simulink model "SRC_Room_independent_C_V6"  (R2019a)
settings: Solver=VariableStepAuto  StartTime=0.0  StopTime=tend  RelTol=1e-6
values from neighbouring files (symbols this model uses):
  initial_switch = zeros(5,1)    [Main_delay.m]
  K_amb = 1    [Main_delay.m]
  K_cw = -10    [Main_delay.m]
  K_eh = 8    [Main_delay.m]
  K_hw = 12    [Main_delay.m]
  K_rw = -5    [Main_delay.m]
  Kc_CW = 1/K_cw*tau_cw/(tauC2+theta_cw)    (= -0.25)    [Main_delay.m]
  Kc_EH = 1/K_eh*tau_eh/(tauC4+theta_eh)    (= 0.3125)    [Main_delay.m]
  Kc_HW = 1/K_hw*tau_hw/(tauC3+theta_hw)    (= 0.138888888889)    [Main_delay.m]
  Kc_RW = 1/K_rw*tau_rw/(tauC1+theta_rw)    (= -0.4)    [Main_delay.m]
  KI_RW = Kc_RW/tau_I_RW    [Main_delay.m]
  Tamb0 = 18    [Main_delay.m]
  Tamb1 = 2    [Main_delay.m]
  Tamb2 = 9    [Main_delay.m]
  Tamb3 = -5    [Main_delay.m]
  Tamb4 = -25    [Main_delay.m]
  Tamb5 = 18    [Main_delay.m]
  Tamb6 = 5    [Main_delay.m]
  tau_amb = 15    [Main_delay.m]
  tau_cw = 15    [Main_delay.m]
  tau_eh = 5    [Main_delay.m]
  tau_hw = 10    [Main_delay.m]
  tau_I_CW = min(tau_cw,4*(tauC2+theta_cw))    [Main_delay.m]
  tau_I_EH = min(tau_eh,4*(tauC4+theta_eh))    [Main_delay.m]
  tau_I_HW = min(tau_hw,4*(tauC3+theta_hw))    [Main_delay.m]
  tau_I_RW = min(tau_rw,4*(tauC1+theta_rw))    [Main_delay.m]
  tau_rw = 8    [Main_delay.m]
  theta_amb = 6    [Main_delay.m]
  theta_cw = 3    [Main_delay.m]
  theta_eh = 1    [Main_delay.m]
  theta_hw = 3    [Main_delay.m]
  theta_rw = 2    [Main_delay.m]
  Tr0 = 18    [Main_delay.m]
  Tsp0 = 18    [Main_delay.m]
  Tsp1 = 0    [Main_delay.m]
  Tsp2 = 0    [Main_delay.m]
  Tsp3 = 0    [Main_delay.m]
  Tsp4 = 0    [Main_delay.m]
  Tt_CW = 1    [Main_delay.m]
  Tt_EH = 1    [Main_delay.m]
  Tt_HW = 1    [Main_delay.m]
  Tt_RW = 1    [Main_delay.m]
  tTamb1 = tTsp1    (= 10)    [Main_delay.m]
  tTamb2 = 80    [Main_delay.m]
  tTamb3 = 140    [Main_delay.m]
  tTamb4 = 180    [Main_delay.m]
  tTamb5 = 280    [Main_delay.m]
  tTamb6 = 350    [Main_delay.m]
  tTsp1 = 10    [Main_delay.m]
  tTsp2 = tTsp1+40    (= 50)    [Main_delay.m]
  tTsp3 = tTsp2+40    (= 90)    [Main_delay.m]
  tTsp4 = tTsp3+40    (= 130)    [Main_delay.m]
  v1max = 1    [Main_delay.m]
  v1min = 0    [Main_delay.m]
  v2max = 1    [Main_delay.m]
  v2min = 0    [Main_delay.m]
  v3max = 1    [Main_delay.m]
  v3min = 0    [Main_delay.m]
  v4max = 1    [Main_delay.m]
  v4min = 0    [Main_delay.m]
libraries: simulink x1

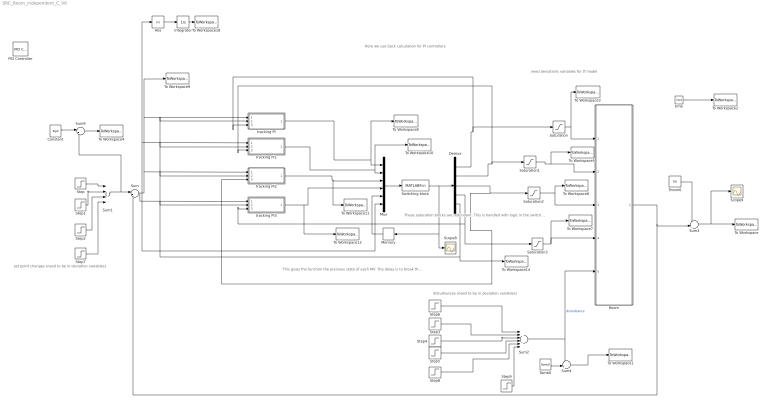
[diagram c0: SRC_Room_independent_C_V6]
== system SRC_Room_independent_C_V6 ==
  note: Here we use back calculation for PI controllers
  note: disturbances (need to be in deviation variables)
  note: set point changes (need to be in deviation variables)
  note: need deviations variables for tf model
  note: This gives the function the preivous state of each MV. The delay is to break the algebraic loop.
  note: These saturation blocks are redundant. This is handled with logic in the switching block.
  Abs : Abs
  Constant : Constant  Value=Tsp0
  Demux : Demux  Outputs=5
  Integrator : Integrator
  Memory : Memory  InitialCondition=initial_switch  InheritSampleTime=on
  Mux : Mux  Inputs=6
  PID Controller : simulink/Continuous/PID Controller  Controller=PI  Form=Parallel  TimeDomain=Continuous-time  SampleTime=-1  IntegratorMethod=Forward Euler  FilterMethod=Forward Euler  ControllerParametersSource=internal  P=Kc_RW  I=KI_RW  D=0  UseFilter=on  N=100  TunerSelectOption=Transfer Function Based (PID Tuner App)  InitialConditionSource=internal  InitialConditionForIntegrator=0  InitialConditionForFilter=0  DifferentiatorICPrevScaledInput=0  ExternalReset=none  TrackingMode=on  Kt=1  LimitOutput=off  UpperSaturationLimit=inf  LowerSaturationLimit=-inf  LinearizeAsGain=on  AntiWindupMode=none  Kb=1  POutMin=[]  POutMax=[]  IOutMin=[]  IOutMax=[]  DOutMin=[]  DOutMax=[]  NOutMin=[]  NOutMax=[]  SumOutMin=[]  SumOutMax=[]  SaturationOutMin=[]  SaturationOutMax=[]  PParamMin=[]  PParamMax=[]  IParamMin=[]  IParamMax=[]  DParamMin=[]  DParamMax=[]  NParamMin=[]  NParamMax=[]  KbParamMin=[]  KbParamMax=[]  KtParamMin=[]  KtParamMax=[]  KbOutMin=[]  KbOutMax=[]  KtOutMin=[]  KtOutMax=[]  IntegratorOutMin=[]  IntegratorOutMax=[]  FilterOutMin=[]  FilterOutMax=[]  SumI1OutMin=[]  SumI1OutMax=[]  SumI2OutMin=[]  SumI2OutMax=[]  SumI3OutMin=[]  SumI3OutMax=[]  SumI4OutMin=[]  SumI4OutMax=[]  SumDOutMin=[]  SumDOutMax=[]  DifferentiatorOutMin=[]  DifferentiatorOutMax=[]  FilterDiffOutCoefMin=[]  FilterDiffOutCoefMax=[]  ReciprocalOutMin=[]  ReciprocalOutMax=[]  SumDenOutMin=[]  SumDenOutMax=[]  SumNumOutMin=[]  SumNumOutMax=[]  DivideOutMin=[]  DivideOutMax=[]  IntegratorContinuousStateAttributes=''  IntegratorStateMustResolveToSignalObject=off  IntegratorRTWStateStorageClass=Auto  FilterContinuousStateAttributes=''  FilterStateMustResolveToSignalObject=off  FilterRTWStateStorageClass=Auto  ParallelPVariant=InternalParameters  IdealPVariant=Disabled  IVariant=InternalParameters  DVariant=Disabled  IntegratorVariant=Continuous  SatVariant=Disabled  AWVariant=Passthrough  PCopyVariant=Disabled  TRVariant=Enabled  FdbkBlocksVariant=Forward  IdealPFdbkVariant=Disabled  SatFdbkVariant=Disabled  DerivativeFilterVariant=Disabled  NVariant=Disabled  NCopyVariant=Disabled_SignalSpec  FilterICVariant=Disabled  IntegratorICVariant=InternalICs  ExternalResetVariant=Disabled  TRSumVariant=TrackingMode  SumFdbkVariant=Disabled  SumVariant=Sum_PI
  Room : Subsystem
  Saturation : Saturate  UpperLimit=v1max  LowerLimit=v1min  ZeroCross=off
  Saturation1 : Saturate  UpperLimit=v2max  LowerLimit=v2min  ZeroCross=off
  Saturation2 : Saturate  UpperLimit=v3max  LowerLimit=v3min  ZeroCross=off
  Saturation3 : Saturate  UpperLimit=v4max  LowerLimit=v4min  ZeroCross=off
  Scope8 : Scope
  Scope9 : Scope
  Step : Step  Time=tTsp1  After=Tsp1  SampleTime=0
  Step1 : Step  Time=tTsp2  After=Tsp2  SampleTime=0
  Step2 : Step  Time=tTsp3  After=Tsp3  SampleTime=0
  Step3 : Step  Time=tTamb2  After=Tamb2  SampleTime=0
  Step4 : Step  Time=tTamb3  After=Tamb3  SampleTime=0
  Step5 : Step  Time=tTamb4  After=Tamb4  SampleTime=0
  Step6 : Step  Time=tTamb1  After=Tamb1  SampleTime=0
  Step7 : Step  Time=tTsp4  After=Tsp4  SampleTime=0
  Step8 : Step  Time=tTamb5  After=Tamb5  SampleTime=0
  Step9 : Step  Time=tTamb6  After=Tamb6  SampleTime=0
  Sum : Sum  Inputs=|+-
  Sum1 : Sum  Inputs=++++
  Sum2 : Sum  Inputs=++++++
  Sum3 : Sum  Inputs=++|
  Sum4 : Sum  Inputs=++|
  Sum9 : Sum  Inputs=|++
  Switching block : MATLABFcn  MATLABFcn=SR7  OutputDimensions=5
  Tamb0 : Constant  Value=Tamb0
  To Workspace : ToWorkspace  VariableName=T  SampleTime=-1
  To Workspace1 : ToWorkspace  VariableName=Tamb  SampleTime=-1
  To Workspace10 : ToWorkspace  VariableName=deltav2  SampleTime=-1
  To Workspace11 : ToWorkspace  VariableName=deltav3  SampleTime=-1
  To Workspace12 : ToWorkspace  VariableName=deltav4  SampleTime=-1
  To Workspace14 : ToWorkspace  VariableName=activeMV  SampleTime=-1
  To Workspace18 : ToWorkspace  VariableName=IAE  SampleTime=-1
  To Workspace2 : ToWorkspace  VariableName=t  SampleTime=-1
  To Workspace3 : ToWorkspace  VariableName=u1  SampleTime=-1
  To Workspace4 : ToWorkspace  VariableName=Tsp  SampleTime=-1
  To Workspace5 : ToWorkspace  VariableName=u2  SampleTime=-1
  To Workspace6 : ToWorkspace  VariableName=u3  SampleTime=-1
  To Workspace7 : ToWorkspace  VariableName=u4  SampleTime=-1
  To Workspace8 : ToWorkspace  VariableName=deltav1  SampleTime=-1
  To Workspace9 : ToWorkspace  VariableName=T_error  SampleTime=-1
  Troom0 : Constant  Value=Tr0
  time : Clock
  tracking PI : Subsystem
  tracking PI1 : Subsystem
  tracking PI2 : Subsystem
  tracking PI3 : Subsystem
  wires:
  Room/1(T) -> Sum3/2, Sum/2  "T"
  Troom0/1 -> Sum3/1
  Sum3/1 -> Scope9/1, To Workspace/1
  Step5/1 -> Sum2/4
  Step4/1 -> Sum2/3
  Step6/1 -> Sum2/1
  Step3/1 -> Sum2/2
  Sum4/1 -> To Workspace1/1
  Tamb0/1 -> Sum4/2
  Constant/1 -> Sum9/1
  Sum1/1 -> Sum9/2, Sum/1
  Step7/1 -> Sum1/4
  Step2/1 -> Sum1/3
  Step/1 -> Sum1/1
  Step1/1 -> Sum1/2
  Sum9/1 -> To Workspace4/1
  Sum/1 -> tracking PI3/1(error), Mux/6, Abs/1, tracking PI1/1(error), tracking PI2/1(error), tracking PI/1(error), To Workspace9/1
  Demux/1 -> tracking PI/3(actual u), Saturation/1
  Demux/2 -> tracking PI1/3(actual u), Saturation1/1
  Demux/3 -> tracking PI2/3(actual u), Saturation2/1
  Demux/4 -> tracking PI3/3(actual u), Saturation3/1
  Saturation1/1 -> To Workspace5/1, Room/2(vCW)
  Saturation2/1 -> Room/3(vHW), To Workspace6/1
  Saturation3/1 -> Room/4(vEH), To Workspace7/1
  time/1 -> To Workspace2/1
  Mux/1 -> Switching block/1
  Switching block/1 -> Scope8/1, Memory/1, Demux/1
  Demux/5 -> To Workspace14/1, tracking PI3/2(active), tracking PI2/2(active), tracking PI1/2(active), tracking PI/2(active)
  Step8/1 -> Sum2/5
  Abs/1 -> Integrator/1
  Integrator/1 -> To Workspace18/1
  Step9/1 -> Sum2/6
  Memory/1 -> Mux/5
  Saturation/1 -> To Workspace3/1, Room/1(vRW)
  Sum2/1 -> Sum4/1, Room/5(Tamb)  "disturbance"
  tracking PI/1(suggested u) -> To Workspace8/1, Mux/1
  tracking PI1/1(suggested u) -> To Workspace10/1, Mux/2
  tracking PI2/1(suggested u) -> To Workspace11/1, Mux/3
  tracking PI3/1(suggested u) -> To Workspace12/1, Mux/4

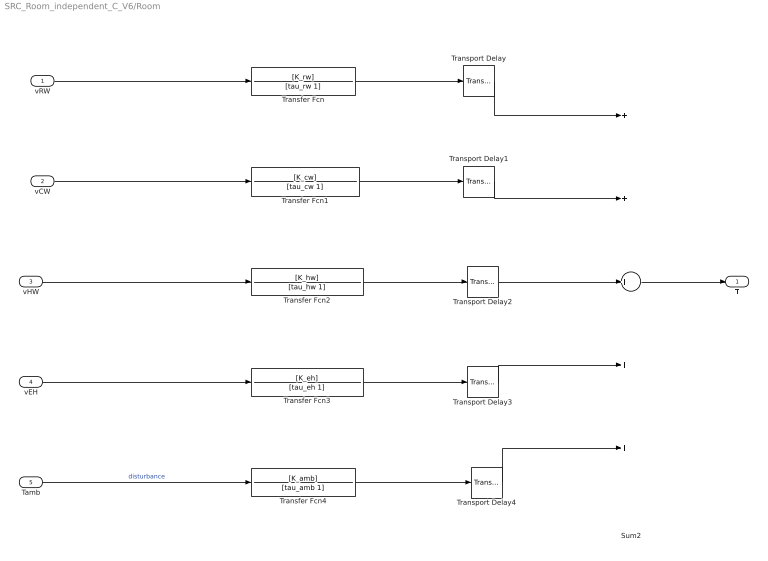
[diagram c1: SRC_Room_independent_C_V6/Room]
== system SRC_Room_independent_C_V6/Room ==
  vRW : Inport
  vCW : Inport  Port=2
  vHW : Inport  Port=3
  vEH : Inport  Port=4
  Tamb : Inport  Port=5
  Sum2 : Sum  Inputs=+++++
  Transfer Fcn : TransferFcn  Numerator=[K_rw]  Denominator=[tau_rw 1]
  Transfer Fcn1 : TransferFcn  Numerator=[K_cw]  Denominator=[tau_cw 1]
  Transfer Fcn2 : TransferFcn  Numerator=[K_hw]  Denominator=[tau_hw 1]
  Transfer Fcn3 : TransferFcn  Numerator=[K_eh]  Denominator=[tau_eh 1]
  Transfer Fcn4 : TransferFcn  Numerator=[K_amb]  Denominator=[tau_amb 1]
  Transport Delay : TransportDelay  DelayTime=theta_rw
  Transport Delay1 : TransportDelay  DelayTime=theta_cw
  Transport Delay2 : TransportDelay  DelayTime=theta_hw
  Transport Delay3 : TransportDelay  DelayTime=theta_eh
  Transport Delay4 : TransportDelay  DelayTime=theta_amb
  T : Outport
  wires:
  vRW/1 -> Transfer Fcn/1
  vCW/1 -> Transfer Fcn1/1
  vHW/1 -> Transfer Fcn2/1
  vEH/1 -> Transfer Fcn3/1
  Sum2/1 -> T/1
  Tamb/1 -> Transfer Fcn4/1  "disturbance"
  Transfer Fcn/1 -> Transport Delay/1
  Transfer Fcn1/1 -> Transport Delay1/1
  Transfer Fcn2/1 -> Transport Delay2/1
  Transfer Fcn3/1 -> Transport Delay3/1
  Transfer Fcn4/1 -> Transport Delay4/1
  Transport Delay/1 -> Sum2/1
  Transport Delay1/1 -> Sum2/2
  Transport Delay2/1 -> Sum2/3
  Transport Delay3/1 -> Sum2/4
  Transport Delay4/1 -> Sum2/5

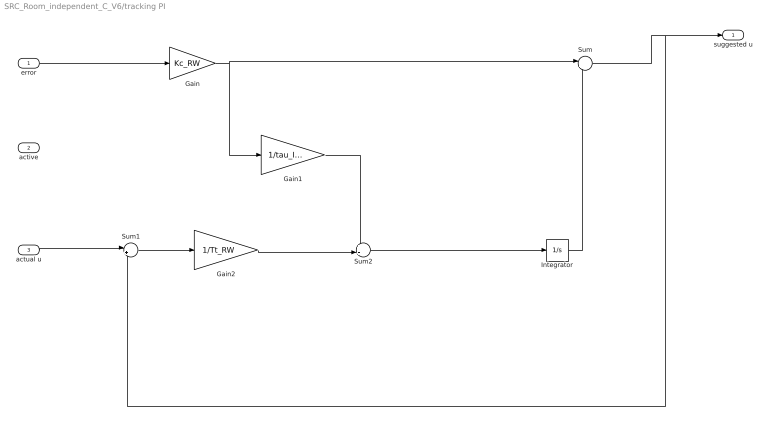
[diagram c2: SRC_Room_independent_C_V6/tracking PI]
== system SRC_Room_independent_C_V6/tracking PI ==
  error : Inport
  active : Inport  Port=2
  actual u : Inport  Port=3
  Gain : Gain  Gain=Kc_RW
  Gain1 : Gain  Gain=1/tau_I_RW
  Gain2 : Gain  Gain=1/Tt_RW
  Integrator : Integrator
  Sum : Sum  Inputs=|++
  Sum1 : Sum  Inputs=|+-
  Sum2 : Sum  Inputs=++|
  suggested u : Outport
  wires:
  Integrator/1 -> Sum/2
  Gain/1 -> Gain1/1, Sum/1
  Sum/1 -> Sum1/2, suggested u/1
  error/1 -> Gain/1
  actual u/1 -> Sum1/1
  Sum1/1 -> Gain2/1
  Gain2/1 -> Sum2/2
  Gain1/1 -> Sum2/1
  Sum2/1 -> Integrator/1

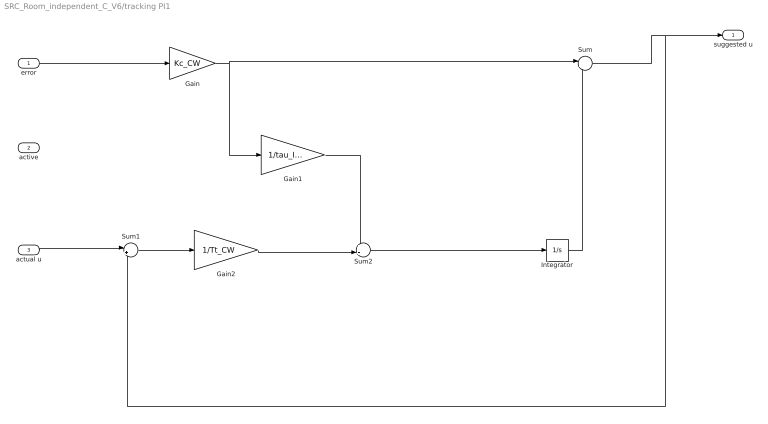
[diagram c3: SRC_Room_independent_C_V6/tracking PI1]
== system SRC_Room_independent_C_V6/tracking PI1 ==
  error : Inport
  active : Inport  Port=2
  actual u : Inport  Port=3
  Gain : Gain  Gain=Kc_CW
  Gain1 : Gain  Gain=1/tau_I_CW
  Gain2 : Gain  Gain=1/Tt_CW
  Integrator : Integrator
  Sum : Sum  Inputs=|++
  Sum1 : Sum  Inputs=|+-
  Sum2 : Sum  Inputs=++|
  suggested u : Outport
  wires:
  Integrator/1 -> Sum/2
  Gain/1 -> Gain1/1, Sum/1
  Sum/1 -> Sum1/2, suggested u/1
  error/1 -> Gain/1
  actual u/1 -> Sum1/1
  Sum1/1 -> Gain2/1
  Gain2/1 -> Sum2/2
  Gain1/1 -> Sum2/1
  Sum2/1 -> Integrator/1

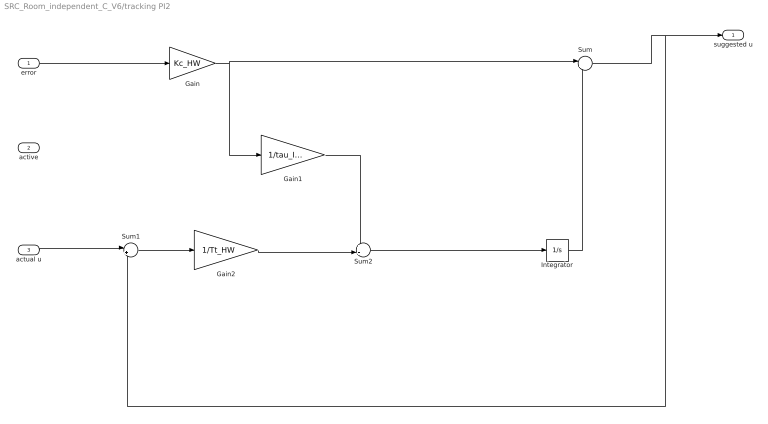
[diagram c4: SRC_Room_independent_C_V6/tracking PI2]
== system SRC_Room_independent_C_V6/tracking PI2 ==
  error : Inport
  active : Inport  Port=2
  actual u : Inport  Port=3
  Gain : Gain  Gain=Kc_HW
  Gain1 : Gain  Gain=1/tau_I_HW
  Gain2 : Gain  Gain=1/Tt_HW
  Integrator : Integrator
  Sum : Sum  Inputs=|++
  Sum1 : Sum  Inputs=|+-
  Sum2 : Sum  Inputs=++|
  suggested u : Outport
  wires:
  Integrator/1 -> Sum/2
  Gain/1 -> Gain1/1, Sum/1
  Sum/1 -> Sum1/2, suggested u/1
  error/1 -> Gain/1
  actual u/1 -> Sum1/1
  Sum1/1 -> Gain2/1
  Gain2/1 -> Sum2/2
  Gain1/1 -> Sum2/1
  Sum2/1 -> Integrator/1

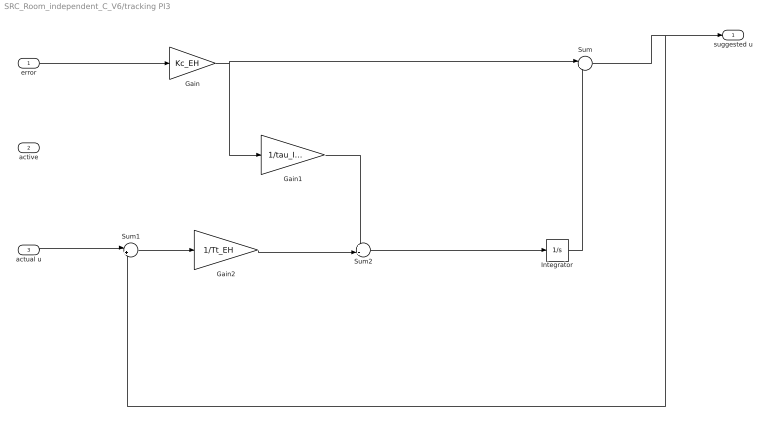
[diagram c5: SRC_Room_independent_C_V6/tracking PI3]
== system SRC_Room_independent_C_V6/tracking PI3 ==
  error : Inport
  active : Inport  Port=2
  actual u : Inport  Port=3
  Gain : Gain  Gain=Kc_EH
  Gain1 : Gain  Gain=1/tau_I_EH
  Gain2 : Gain  Gain=1/Tt_EH
  Integrator : Integrator
  Sum : Sum  Inputs=|++
  Sum1 : Sum  Inputs=|+-
  Sum2 : Sum  Inputs=++|
  suggested u : Outport
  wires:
  Integrator/1 -> Sum/2
  Gain/1 -> Gain1/1, Sum/1
  Sum/1 -> Sum1/2, suggested u/1
  error/1 -> Gain/1
  actual u/1 -> Sum1/1
  Sum1/1 -> Gain2/1
  Gain2/1 -> Sum2/2
  Gain1/1 -> Sum2/1
  Sum2/1 -> Integrator/1
